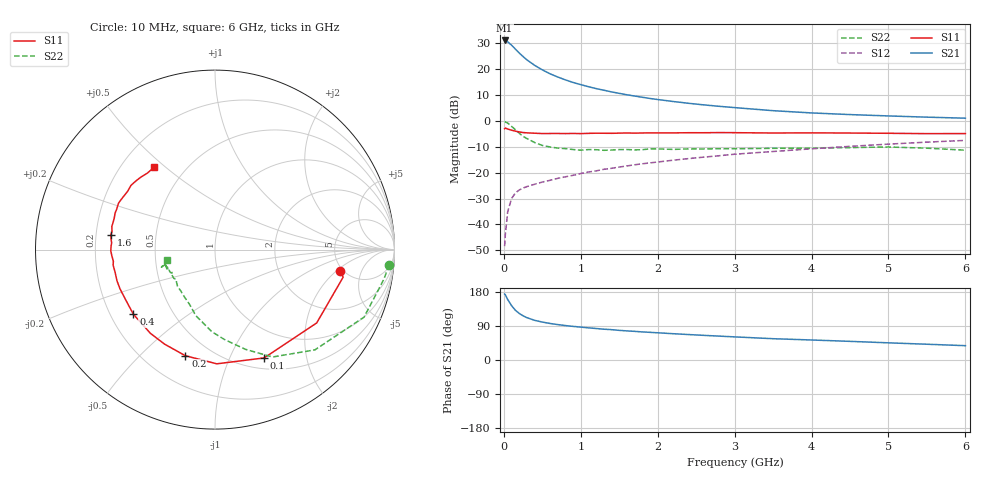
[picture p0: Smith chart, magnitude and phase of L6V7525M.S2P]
!  INFINEON TECHNOLOGIES Small Signal Semiconductors
! BFR380L3 , Si-NPN RF-Transistor in TSLP-3-1
!  Vce=0.75 V,  Ic=25 mA
! Common Emitter S-Parameters:  07. March 2005
#  GHz  S  MA  R  50
! f  S11  S21  S12  S22
! GHz  Mag  Ang  Mag  Ang  Mag  Ang  Mag  Ang
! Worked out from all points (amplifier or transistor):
!   36 points, 10 MHz to 6 GHz, reference 50 ohm
!   highest |S21| = 31.1 dB at 10 MHz (marker M1)
!   |S21| within 3 dB of that: start of sweep to 138.9 MHz
!   unconditionally stable (mu >= 1): 1.591 GHz to 5.614 GHz
!   at 250 MHz: K = 0.42, MSG = 25.4 dB, |S12| = -25.9 dB
!   at 1.4 GHz: K = 0.98, MSG = 14.8 dB, |S12| = -18.3 dB
!   at 6 GHz: K = 1.00, MSG = 4.3 dB, |S12| = -7.5 dB
!   S11 on the Smith chart (normalised r, x): 10 MHz: 4.68, -2.28; 100 MHz: 0.63, -1.35; 200 MHz: 0.37, -0.69; 400 MHz: 0.30, -0.32; 1.6 GHz: 0.26, +0.07; 6 GHz: 0.34, +0.46
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0.01  0.7073 -9.9  36.01 174.1  0.0038 79.6  0.9745 -5.0
0.02  0.7304 -12.1  35.71 171.9  0.0065 86.8  0.9547 -10.1
0.05  0.6986 -35.8  33.9 159.7  0.0176 74.7  0.9116 -24.4
0.1  0.6628 -65.6  29.21 143.5  0.0316 62.8  0.7887 -45.1
0.15  0.6364 -89.1  24.52 131.3  0.0405 54.4  0.6789 -61.8
0.2  0.6139 -105.6  20.59 122.8  0.0463 51.2  0.5812 -73.0
0.25  0.597 -118.0  17.6 116.6  0.0505 48.6  0.5031 -84.1
0.3  0.5892 -127.6  15.18 111.7  0.0539 47.4  0.4582 -92.1
0.4  0.5801 -141.6  11.91 104.7  0.0598 47.5  0.3827 -106.3
0.5  0.5709 -150.9  9.741 100.1  0.0659 49.0  0.3365 -114.9
0.6  0.5726 -157.6  8.168 96.4  0.0712 50.3  0.3146 -122.6
0.7  0.5731 -162.3  7.082 93.5  0.0777 52.1  0.2991 -129.6
0.9  0.5742 -171.3  5.549 88.7  0.089 55.4  0.2803 -140.1
1.1  0.5761 -176.7  4.596 84.8  0.103 57.4  0.2801 -145.1
1.3  0.5792 177.9  3.927 81.3  0.1163 58.7  0.2708 -152.0
1.6  0.5862 171.8  3.209 76.8  0.1352 60.1  0.2807 -157.0
2.2  0.5881 162.7  2.381 69.4  0.1744 61.4  0.2819 -159.3
2.8  0.5965 154.4  1.92 63.0  0.213 61.7  0.2903 -163.5
3.5  0.5852 146.1  1.581 56.2  0.257 59.8  0.2962 -162.8
4.5  0.5845 139.7  1.329 49.2  0.3232 58.0  0.3059 -162.4
5.5  0.5689 131.5  1.185 41.6  0.3896 53.8  0.2976 -163.6
6  0.5706 126.3  1.132 37.8  0.4215 51.6  0.2725 -168.1
